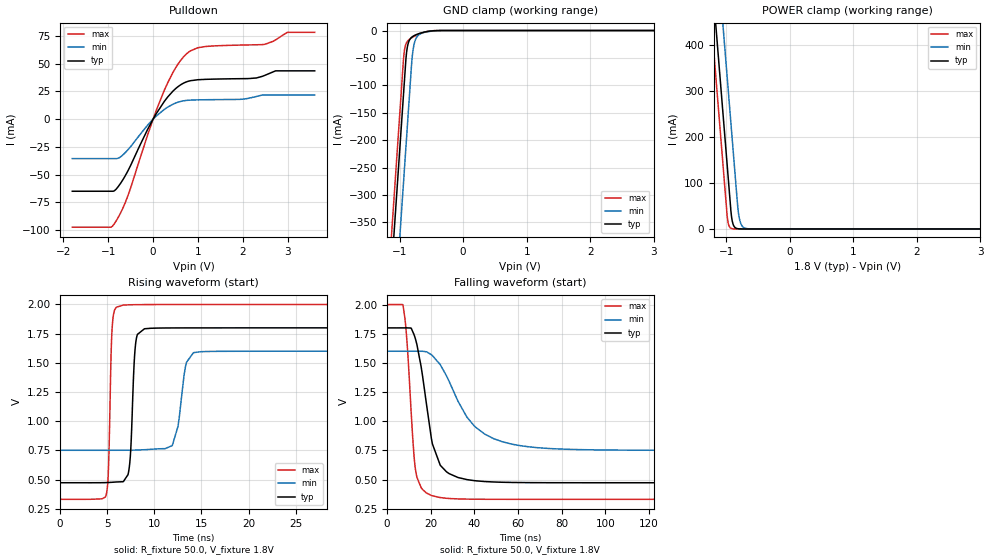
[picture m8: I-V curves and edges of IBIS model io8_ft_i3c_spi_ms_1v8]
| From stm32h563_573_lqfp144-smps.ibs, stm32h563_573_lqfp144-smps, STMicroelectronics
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[Model]   io8_ft_i3c_spi_ms_1v8
Model_type I/O_open_drain
Polarity   Non-Inverting
Enable   Active-Low
| CAP_THRESHOLD on pad IOFT is "UDTCAPC" :
| Rising=20.0% of vddiom   Falling=80.0% of vddiom
| C_comp min and max val. don't necessarily correlate with the min and max pvt
| but are the smallest and greatest pad capacitance found.
| var   typ   min   max
C_comp   3.75296pF  3.68867pF  3.87697pF
|C_comp_pulldown   3.75296pF  3.68867pF  3.87697pF
Vinl = 800.0mV
Vinh = 1.0V
Vmeas = 900.0mV   | Reference voltage for timing measurements
Cref  = 50.0pF   | Timing specification test load capacitance value
Rref  = 1.0MOhm   | Timing specification test load resistance value
Vref  = 990.0mV   | Timing specification test load voltage
[Model Spec]
| TIME_THRESHOLD on pin ZII2CV11 is "CMOS" :
| Rising=40.0% of vdd   Falling=60.0% of vdd
Vinl 703.80000mV 631.80000mV 784.80000mV
Vinh 1.06220V 937.20000mV 1.16620V
| variable   typ   min   max
[Temperature Range] 25.0 125.0 -40.0
| variable   typ   min   max
[Voltage Range] 1.8V 1.6V 2.0V
| variable   typ   min   max
[POWER Clamp Reference] 1.8V 1.6V 2.0V
| variable   typ   min   max
[GND Clamp Reference] 0V 0V 0V
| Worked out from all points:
|   slope of the pulldown table from 0 to 0.27 V, typ, clamps not added: 15.8 ohm
|   GND clamp passes 1 mA (typ) near -0.52 V on its own axis
|   POWER clamp passes 1 mA (typ) near -0.84 V on its own axis
|   rising waveform, R_fixture 50.0, V_fixture 1.8V: 20-80 % time 403ps typ, 844ps min, 285ps max; typ from 0.474 V to 1.8 V
|   falling waveform, R_fixture 50.0, V_fixture 1.8V: 20-80 % time 7.17ns typ, 16.5ns min, 3.35ns max; typ from 1.8 V to 0.474 V
[POWER Clamp]
-1.8V     1.518A     1.709A     1.407A
-1.23V    548.8mA    740.2mA    437.5mA
-1.16V    429.8mA    621.2mA    318.5mA
-1.05V    242.8mA    434.2mA    131.5mA
-980mV    123.8mA    315.2mA    17.95mA
-930mV    38.81mA    230.2mA    1.49mA
-910mV    17.82mA    196.2mA    550.8uA
-890mV    8.18mA     162.2mA    203.5uA
-810mV    363.5uA    33.6mA     3.797uA
-770mV    76.62uA    10.47mA    518.8nA
-710mV    7.416uA    1.822mA    26.34nA
3.6V      0A         0A         0A
[GND Clamp]
-1.8V     -1.579A    -1.74A     -1.515A
-1.24V    -627.3mA   -788.3mA   -562.7mA
-1.05V    -304.3mA   -465.3mA   -239.7mA
-940mV    -117.3mA   -278.3mA   -52.69mA
-930mV    -100.3mA   -261.3mA   -40.52mA
-900mV    -50.11mA   -210.3mA   -24.23mA
-880mV    -30.95mA   -176.3mA   -20.02mA
-810mV    -12.18mA   -57.97mA   -13.23mA
-780mV    -9.807mA   -29.1mA    -11.19mA
-690mV    -5.41mA    -7.142mA   -6.184mA
-420mV    -170.4uA   -446.1uA   -81.94uA
3.6V      5.755nA    953.4nA    228.2pA
| variable   typ   min   max
[Pullup Reference] 1.8V 1.6V 2.0V
| variable   typ   min   max
[Pulldown Reference] 0V 0V 0V
[Pulldown]
-1.8V     -65.02mA   -35.56mA   -97.42mA
-940mV    -65.02mA   -35.56mA   -97.42mA
-850mV    -64.17mA   -35.56mA   -93.49mA
-570mV    -47.32mA   -28.01mA   -70.04mA
-120mV    -9.088mA   -5.279mA   -14.07mA
250mV     16.04mA    8.832mA    26.05mA
520mV     28.19mA    14.82mA    47.53mA
780mV     34.17mA    17.07mA    60.14mA
1.18V     35.97mA    17.56mA    65.65mA
2.49V     39.57mA    21.77mA    67.55mA
2.99V     43.62mA    21.77mA    78.38mA
3.6V      43.62mA    21.77mA    78.38mA
[Ramp]
dV/dt_r 795.7613mV/399.70706ps 508.92865mV/789.08759ps 1.00097V/282.80702ps
dV/dt_f 795.7872mV/6.62517ns 508.97375mV/16.23004ns 1.00099V/3.34797ns
R_load = 50.0
| Removed startup time: 0s 0s 0s  .
| Removed end time: 36.4ns.
[Rising Waveform]
R_fixture   = 50.0
V_fixture   = 1.8V
V_fixture_min = 1.6V
V_fixture_max = 2.0V
0s        473.7mV    751.7mV    331.7mV
4.85ns    474.9mV    751.7mV    361.7mV
5.5ns     477.5mV    751.8mV    1.774V
5.95ns    480.1mV    751.8mV    1.977V
7.25ns    561mV      752.3mV    1.997V
8ns       1.658V     753.4mV    1.998V
8.95ns    1.792V     756.5mV    1.999V
11.9ns    1.799V     792.1mV    2V
14.15ns   1.8V       1.587V     2V
36.4ns    1.8V       1.6V       2V
| Removed startup time: 0s 0s 0s  .
| Removed end time: 199.4ns.
[Falling Waveform]
R_fixture   = 50.0
V_fixture   = 1.8V
V_fixture_min = 1.6V
V_fixture_max = 2.0V
0s        1.8V       1.6V       2V
7.3ns     1.8V       1.6V       1.996V
9.1ns     1.8V       1.6V       1.699V
11.7ns    1.772V     1.6V       887mV
13.05ns   1.705V     1.6V       586.3mV
20.35ns   851.7mV    1.57V      364.8mV
28.5ns    551.6mV    1.341V     338.8mV
39.8ns    492.1mV    963.9mV    332.8mV
57ns      476.4mV    804.9mV    331.7mV
199.4ns   473.7mV    751.7mV    331.7mV
